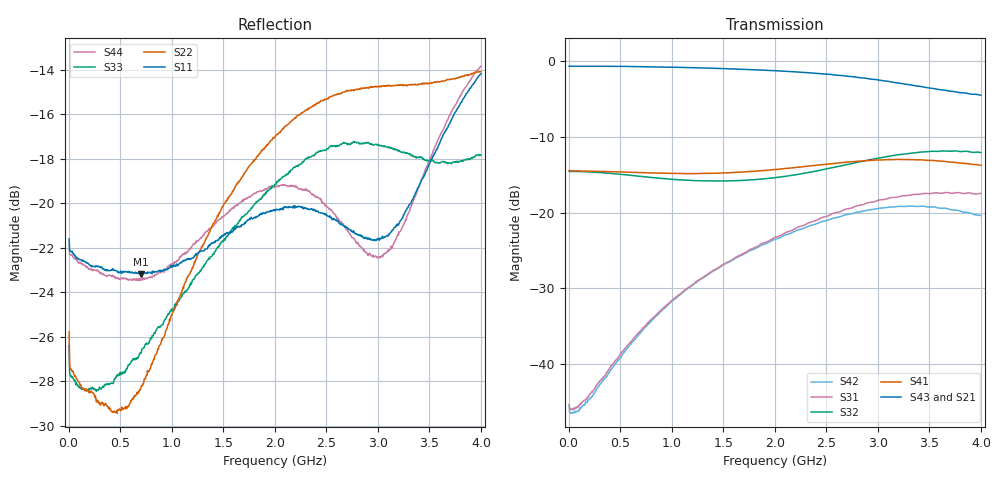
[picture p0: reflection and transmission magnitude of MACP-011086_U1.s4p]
!Agilent Technologies,E5071C,MY46110647,A.11.31
!Date: Thu Jul 09 12:03:04 2020 DD
!Data & Calibration Information:
!MACP-011086 soldered onto PT-0010289 with SMA connectors, calibration PCB PT-0003654. Port1 (pin1) Port2 (pin5) Port3 (pin4) Port4 (pin3)
!Freq	S11:SOLT4(ON)	S12:SOLT4(ON)	S13:SOLT4(ON)	S14:SOLT4(ON)
!	S21:SOLT4(ON)	S22:SOLT4(ON)	S23:SOLT4(ON)	S24:SOLT4(ON)
!	S31:SOLT4(ON)	S32:SOLT4(ON)	S33:SOLT4(ON)	S34:SOLT4(ON)
!	S41:SOLT4(ON)	S42:SOLT4(ON)	S43:SOLT4(ON)	S44:SOLT4(ON)
!PortZ  Port1:50+j0  Port2:50+j0  Port3:50+j0  Port4:50+j0
!Above PortZ is port z conversion or system Z0 setting when saving the data.
!When reading, reference impedance value at option line is always used.
# Hz S MA R 50
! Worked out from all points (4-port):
!   800 points, 5 MHz to 4 GHz, reference 50 ohm
!   strongest paths, dB at 5 MHz, 1.005 GHz, 2.005 GHz, 3.005 GHz, 4 GHz:
!     S43: -0.7, -0.8, -1.3, -2.5, -4.5
!     S21: -0.7, -0.8, -1.3, -2.5, -4.3
!     S41: -14.5, -14.8, -14.3, -13.1, -13.8
!     S32: -14.6, -15.6, -15.4, -12.8, -12.1
!     S31: -45.3, -31.6, -23.3, -18.4, -17.5
!     S42: -45.3, -31.7, -23.5, -19.5, -20.4
!   lowest |S11| = -23.2 dB at 705 MHz (marker M1), VSWR 1.15, Z = 47.7 + j6.38 ohm
!   |S11| at or under -10 dB: start of sweep to end of sweep
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5000000  0.08322 160.0  0.9212 1.6  0.005702 166.8  0.1895 -179.0
         0.9207 1.6  0.05141 145.1  0.1863 1.8  0.005176 174.1
         0.005424 171.0  0.1867 1.8  0.04793 146.9  0.9215 1.3
         0.1894 -179.2  0.005407 178.1  0.922 1.4  0.08076 162.5
4.3e8  0.07136 134.9  0.9202 -10.7  0.01008 172.5  0.186 153.4
       0.9202 -10.7  0.03393 114.5  0.1805 -7.8  0.009733 170.2
       0.01007 173.1  0.1806 -7.8  0.03935 112.3  0.9202 -11.1
       0.1858 153.4  0.009596 170.5  0.9203 -11.1  0.0689 131.1
7.05e8  0.06938 106.2  0.916 -17.7  0.0164 153.4  0.1835 137.1
        0.9163 -17.7  0.03878 68.5  0.1731 -11.2  0.0163 151.4
        0.0168 153.0  0.1731 -11.3  0.04611 78.5  0.9156 -18.3
        0.1834 137.2  0.01638 151.9  0.9158 -18.3  0.06743 99.2
1.51e9  0.08501 33.0  0.8881 -38.2  0.04483 98.3  0.1827 93.9
        0.8885 -38.2  0.09994 -2.6  0.162 -14.0  0.04501 97.9
        0.04598 98.5  0.1615 -14.1  0.08278 11.9  0.8888 -39.4
        0.1825 94.1  0.04556 97.9  0.8888 -39.4  0.09381 19.7
2.345e9  0.09718 -6.9  0.8311 -60.0  0.08644 47.3  0.2034 49.0
         0.8313 -59.9  0.1645 -30.9  0.1855 -15.6  0.08097 48.6
         0.08644 48.1  0.1846 -15.7  0.1271 -30.3  0.8342 -62.3
         0.2031 49.4  0.08193 48.9  0.8329 -62.3  0.1058 -17.0
3.04e9  0.08351 0.4  0.7439 -78.0  0.1242 -2.0  0.2227 3.8
        0.7443 -78.0  0.1835 -45.9  0.2331 -27.6  0.1055 2.6
        0.1216 -0.5  0.2308 -27.7  0.1345 -56.4  0.7434 -81.7
        0.2224 4.5  0.107 3.4  0.7402 -81.7  0.07579 1.5
4e9  0.1958 6.5  0.6113 -96.9  0.1383 -81.2  0.2049 -68.2
     0.6077 -96.9  0.1978 -56.9  0.2508 -62.0  0.09434 -69.3
     0.1336 -79.5  0.2483 -61.9  0.1287 -62.7  0.5978 -102.2
     0.205 -67.6  0.0956 -67.9  0.5932 -102.0  0.2035 17.4
